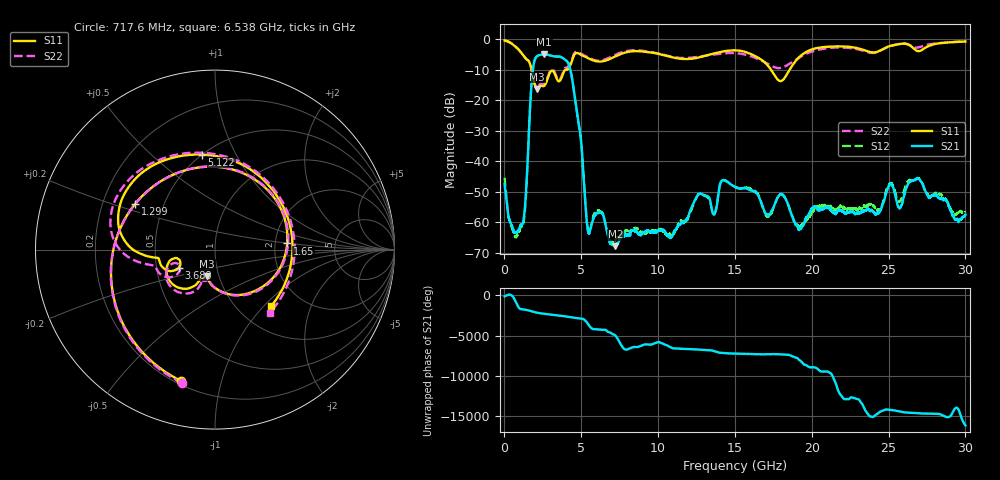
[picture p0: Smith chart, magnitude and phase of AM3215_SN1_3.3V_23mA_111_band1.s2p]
!Agilent Technologies,E8364B,MY43040894,A.07.50.67
!Agilent E8364B: A.07.50.67
!Date: Tuesday, May 25, 2021 15:11:41
!Correction: S11(Full 2 Port(1,2))
!S21(Full 2 Port(1,2))
!S12(Full 2 Port(1,2))
!S22(Full 2 Port(1,2))
!S2P File: Measurements: S11, S21, S12, S22:
# Hz S  dB  R 50
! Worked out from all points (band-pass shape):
!   6401 points, 10 MHz to 30 GHz, reference 50 ohm
!   highest |S21| = -4.98 dB at 2.578 GHz (marker M1); lowest = -67.8 dB at 7.222 GHz (marker M2)
!   |S21| within 3 dB of the highest: 1.91 GHz to 4.164 GHz (2.254 GHz wide, 74.2 % of centre)
!   lowest |S11| = -16.3 dB at 2.123 GHz (marker M3), VSWR 1.36, Z = 43.9 - j13.2 ohm
!   |S11| at or under -10 dB: 1.761 GHz to 4.053 GHz (2.291 GHz wide, 78.8 % of centre); 17.35 GHz to 18.56 GHz (1.21 GHz wide, 6.74 % of centre)
!   |S22| runs from -15.8 to -0.4 dB; largest |S21 - S12| = 0.0063
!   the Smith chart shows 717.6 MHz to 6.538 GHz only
!   S11 on the Smith chart (normalised r, x): 717.6 MHz: 0.22, -0.75; 1.299 GHz: 0.34, +0.24; 1.65 GHz: 2.33, +0.19; 3.688 GHz: 0.65, -0.14; 5.122 GHz: 0.50, +0.74; 6.538 GHz: 1.40, -1.10
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1e7  -0.40 -10.0  -47.42 -119.4  -45.40 -93.4  -0.45 -10.1
7.175766e8  -2.44 -104.6  -63.31 -18.4  -64.71 -111.9  -2.33 -103.9
1.298633e9  -5.80 150.4  -56.83 39.6  -57.88 -140.7  -5.81 150.7
1.650078e9  -7.88 4.9  -24.05 -116.1  -24.11 -115.8  -7.76 5.5
2.123358e9  -16.30 -106.9  -5.55 1.3  -5.54 1.3  -15.80 -102.3
2.577894e9  -15.32 -117.3  -4.98 -132.6  -4.96 -132.7  -14.67 -114.2
3.149578e9  -10.37 -151.5  -5.55 97.5  -5.55 97.3  -9.92 -146.2
3.688461e9  -12.93 -153.6  -5.87 -21.9  -5.87 -22.0  -12.47 -147.9
5.009895e9  -5.14 108.8  -34.57 -12.1  -34.71 -12.2  -4.81 114.3
5.122358e9  -5.44 97.8  -43.12 -57.4  -42.52 -38.3  -5.12 103.2
5.478489e9  -6.30 63.5  -63.54 -83.6  -63.06 -42.1  -6.04 67.5
6.537511e9  -7.07 -45.3  -59.93 37.2  -59.66 17.8  -6.64 -49.0
7.221658e9  -5.62 -110.4  -67.80 19.4  -65.64 30.8  -5.06 -115.0
8.332225e9  -3.93 162.8  -62.56 10.4  -62.13 69.2  -3.64 161.6
1.000979e10  -4.78 49.2  -62.85 -38.1  -62.74 153.3  -4.66 49.3
1.190291e10  -6.49 -92.1  -58.62 161.0  -59.22 161.8  -6.14 -93.2
1.335555e10  -5.02 163.9  -52.25 12.1  -52.93 13.0  -5.16 168.9
1.5005e10  -3.63 65.6  -48.35 -48.4  -48.49 -47.8  -4.54 68.2
1.709024e10  -8.33 -53.6  -57.46 -133.9  -58.00 140.8  -7.93 -78.0
2.00049e10  -3.35 32.1  -55.52 43.4  -57.13 -141.7  -4.04 52.7
2.500479e10  -2.35 -59.8  -48.05 163.9  -47.62 161.5  -2.42 -57.3
3e10  -0.73 -119.4  -57.43 2.2  -56.76 121.3  -0.76 -120.0
